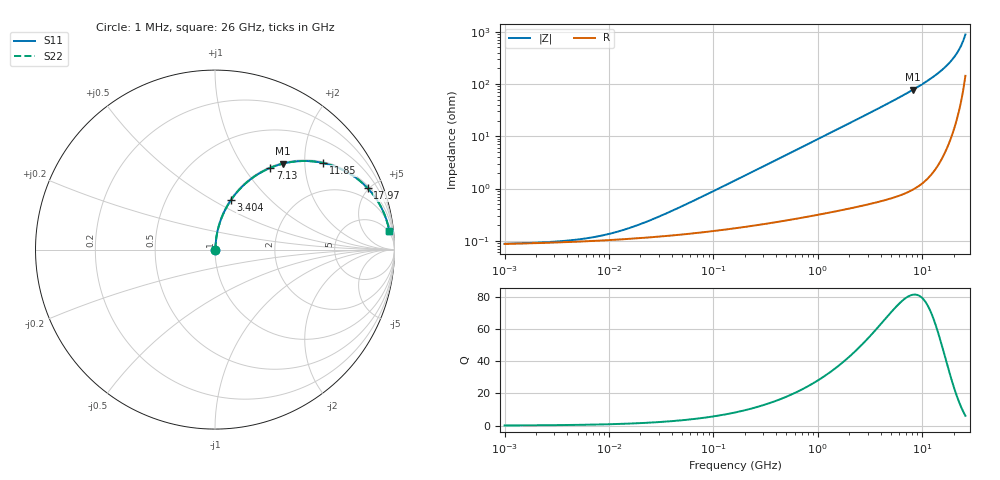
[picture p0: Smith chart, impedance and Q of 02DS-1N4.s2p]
# MHz S MA R 50
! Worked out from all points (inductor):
!   221 points, 1 MHz to 26 GHz, reference 50 ohm
!   read as one part in series: L = 1.4 nH near 44.22 MHz
!   highest Q = 81.1 at 8.19 GHz (marker M1), where L = 1.51 nH
!   S11 on the Smith chart (normalised r, x): 1 MHz: 1.00, +0.00; 3.404 GHz: 1.01, +0.61; 7.13 GHz: 1.02, +1.33; 11.85 GHz: 1.03, +2.47; 17.97 GHz: 1.14, +4.91; 26 GHz: 4, +18
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1  0.0008776 5.7  0.9991 -0.0  0.9991 -0.0  0.0008776 5.7
2.76374  0.0009536 14.7  0.9991 -0.0  0.9991 -0.0  0.0009536 14.7
5.52737  0.001088 26.5  0.999 -0.0  0.999 -0.0  0.001088 26.5
8.37782  0.001252 36.0  0.999 -0.0  0.999 -0.0  0.001252 36.0
12.6982  0.001541 46.3  0.9989 -0.1  0.9989 -0.1  0.001541 46.3
19.2467  0.00203 56.3  0.9989 -0.1  0.9989 -0.1  0.00203 56.3
30.5518  0.002943 65.6  0.9988 -0.2  0.9988 -0.2  0.002943 65.6
168.871  0.01493 82.4  0.9981 -0.8  0.9981 -0.8  0.01493 82.4
891.261  0.07805 83.3  0.994 -4.5  0.994 -4.5  0.07805 83.3
1782.48  0.1549 79.7  0.9841 -8.9  0.9841 -8.9  0.1549 79.7
3403.91  0.2889 72.2  0.9524 -16.8  0.9524 -16.8  0.2889 72.2
4926.33  0.4047 65.3  0.9087 -23.9  0.9087 -23.9  0.4047 65.3
7129.64  0.5503 55.9  0.8281 -33.4  0.8281 -33.4  0.5503 55.9
8189.77  0.6105 51.7  0.7846 -37.6  0.7846 -37.6  0.6105 51.7
9852.45  0.6922 45.5  0.713 -43.8  0.713 -43.8  0.6922 45.5
11852.7  0.7717 38.7  0.6253 -50.5  0.6253 -50.5  0.7717 38.7
14933.3  0.8604 29.6  0.4937 -59.3  0.4937 -59.3  0.8604 29.6
17965.1  0.9169 21.9  0.3736 -66.4  0.3736 -66.4  0.9169 21.9
20636.4  0.9482 16.1  0.2771 -71.3  0.2771 -71.3  0.9482 16.1
22634.4  0.9632 12.1  0.2108 -73.9  0.2108 -73.9  0.9632 12.1
24825.9  0.9732 8.2  0.1436 -75.2  0.1436 -75.2  0.9732 8.2
26000  0.9762 6.2  0.1101 -74.4  0.1101 -74.4  0.9762 6.2
